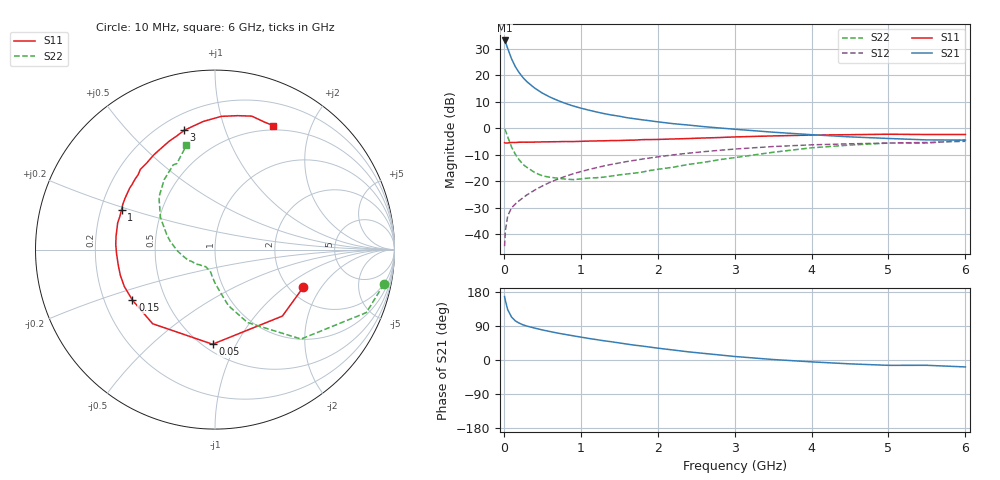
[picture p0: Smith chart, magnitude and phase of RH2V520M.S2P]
! SIEMENS Small Signal Semiconductors
! BFR106
! Si NPN RF Bipolar Junction Transistor in SOT23
! VCE = 2.5 V  IC = 20 mA
! Common Emitter S-Parameters:  August  1996
# GHz  S  MA  R  50
!  f  S11  S21  S12  S22
! GHz  MAG  ANG  MAG  ANG  MAG  ANG  MAG  ANG
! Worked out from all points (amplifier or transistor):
!   36 points, 10 MHz to 6 GHz, reference 50 ohm
!   highest |S21| = 33.1 dB at 10 MHz (marker M1)
!   |S21| within 3 dB of that: start of sweep to 50.13 MHz
!   unconditionally stable (mu >= 1): 358.1 MHz to 2.385 GHz; 5.203 GHz to end of sweep
!   at 250 MHz: K = 0.90, MSG = 22.6 dB, |S12| = -26.2 dB
!   at 1.4 GHz: K = 1.07, MAG = 7.6 dB, |S12| = -13.6 dB
!   at 6 GHz: K = 1.01, MAG = -0.4 dB, |S12| = -4.9 dB
!   S11 on the Smith chart (normalised r, x): 10 MHz: 2.36, -1.39; 50 MHz: 0.55, -0.81; 150 MHz: 0.32, -0.25; 1 GHz: 0.29, +0.19; 3 GHz: 0.29, +0.73; 6 GHz: 0.45, +1.48
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0.01  0.5345 -23.2  45.12 167.4  0.006 83.4  0.9604 -11.6
0.02  0.5274 -44.6  42.52 156.9  0.0116 71.6  0.9132 -22.6
0.05  0.5274 -91.5  31.98 132.9  0.0223 58.3  0.6916 -46.1
0.1  0.5398 -130.1  20.39 113.4  0.0316 51.1  0.4447 -66.0
0.15  0.5393 -148.5  14.42 103.1  0.0375 52.2  0.3224 -76.4
0.2  0.5454 -157.7  11.13 97.3  0.0432 54.6  0.2534 -81.6
0.25  0.5465 -164.8  8.969 92.7  0.0491 57.1  0.2079 -86.6
0.3  0.5458 -169.8  7.536 89.5  0.0555 59.3  0.1836 -90.4
0.4  0.5488 -177.3  5.728 84.2  0.0682 62.2  0.1469 -96.6
0.5  0.5537 177.1  4.601 79.4  0.0817 64.1  0.1271 -101.2
0.6  0.5562 172.3  3.865 75.1  0.096 64.5  0.1189 -105.1
0.8  0.5623 164.6  2.943 67.4  0.1241 64.5  0.1103 -115.3
1  0.5667 156.8  2.394 60.5  0.1524 63.4  0.111 -122.1
1.1  0.5728 153.5  2.201 57.0  0.1662 62.4  0.1151 -127.0
1.3  0.5804 147.5  1.891 50.8  0.1948 60.3  0.1198 -135.1
1.6  0.5939 138.5  1.582 42.0  0.236 56.6  0.1375 -147.1
2.2  0.6283 122.9  1.221 26.4  0.3147 48.2  0.1844 -169.7
3  0.6864 104.5  0.959 9.3  0.4058 35.5  0.2794 163.3
3.5  0.7171 95.2  0.843 1.3  0.4525 27.8  0.3528 149.5
4.5  0.7569 80.4  0.688 -10.2  0.509 12.6  0.4822 125.9
5.5  0.7622 68.9  0.603 -14.0  0.5395 3.0  0.5245 113.9
6  0.763 64.9  0.598 -18.3  0.5678 -4.1  0.6028 105.3
